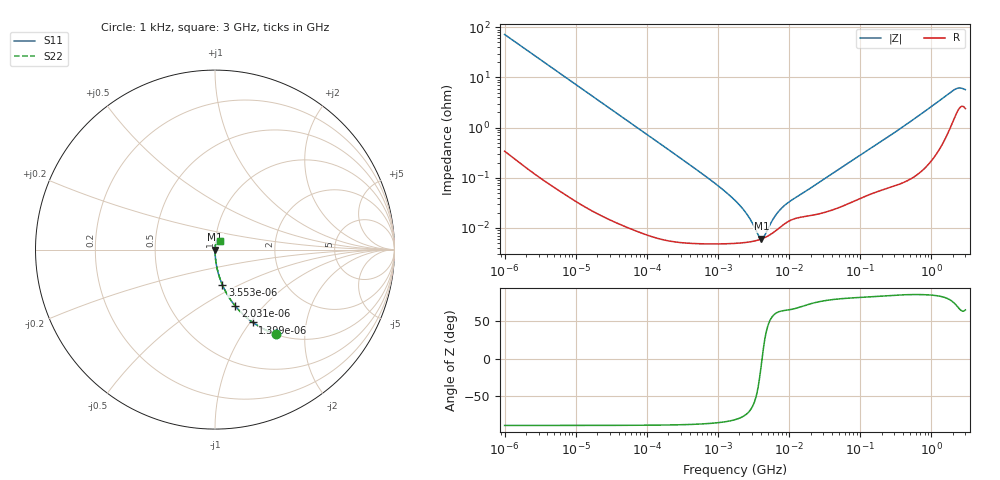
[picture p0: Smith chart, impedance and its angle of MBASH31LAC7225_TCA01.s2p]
! MBASH31LAC7225_TCA01  S-PARAMETER MODEL  ( Standard Model )
! Model Generated by TAIYO YUDEN Corporation (http://www.ty-top.com)
! Version 1.0
! TAIYO YUDEN Control No. 220601
! Copyright(c) 2016 TAIYO YUDEN CO.,LTD. All Rights Reserved.
! Product Description (link to TY-COMPAS)
! https://ds.yuden.co.jp/TYCOMPAS/or/detail?pn=MBASH31LAC7225KTCA01&u=M
! Products Name : Multilayer Ceramic Capacitors
! Characteristics :
!  Capacitance : 2.2 [uF] , Rated Voltage : 100 [V] , TCC : X7S
!  Case Size : 3.2 x 1.6 / 0.126 x 0.063 [mm/inch] , Thickness : 1.6 / 0.063 [mm/inch]
!  (Conditions: Temperature = 25 [degC] , DC Bias Voltage = 0 [V])
! External Node Assignments :
!  1  o---| |---o  2
! GND o---------o GND
! Frequency Range : 1kHz  -  3GHz  [ 401 STEP ]
# MHZ S RI R 50
! Freq[MHz].  S11 Real  S11 Imag  S21 Real  S21 Imag  S12 Real  S12 Imag  S22 Real  S22 Imag
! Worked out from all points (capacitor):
!   401 points, 1 kHz to 3 GHz, reference 50 ohm
!   read as one part in series: C = 2.21 uF near 1.077 kHz
!   lowest |Z| = 6.02 mohm at 4.083 MHz (marker M1)
!   series resonance near 4.159 MHz, so ESL is about 660 pH
!   S11 on the Smith chart (normalised r, x): 1 kHz: 1.01, -1.44; 1.399 kHz: 1.00, -1.03; 2.031 kHz: 1.00, -0.71; 3.553 kHz: 1.00, -0.41; 3 GHz: 1.05, +0.10
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0.001  0.3423 -0.4721  0.6577 0.4721  0.6577 0.4721  0.3423 -0.4721
0.001399  0.211 -0.4057  0.789 0.4057  0.789 0.4057  0.211 -0.4057
0.002031  0.1132 -0.3147  0.8868 0.3147  0.8868 0.3147  0.1132 -0.3147
0.003553  0.0405 -0.195  0.9595 0.195  0.9595 0.195  0.0405 -0.195
0.006215  0.0139 -0.1148  0.9861 0.1148  0.9861 0.1148  0.0139 -0.1148
0.01216  0.00382 -0.0594  0.9962 0.0594  0.9962 0.0594  0.00382 -0.0594
0.147855  8.47e-05 -0.00493  0.9999 0.00493  0.9999 0.00493  8.47e-05 -0.00493
0.791611  4.84e-05 -0.00089  1 0.00089  1 0.00089  4.84e-05 -0.00089
1.732051  4.89e-05 -0.000349  1 0.000349  1 0.000349  4.89e-05 -0.000349
2.422679  5.09e-05 -0.0002  0.9999 0.0002  0.9999 0.0002  5.09e-05 -0.0002
3.264662  5.46e-05 -8.61e-05  0.9999 8.61e-05  0.9999 8.61e-05  5.46e-05 -8.61e-05
3.517417  5.6e-05 -5.92e-05  0.9999 5.92e-05  0.9999 5.92e-05  5.6e-05 -5.92e-05
4.083148  5.99e-05 -6.44e-06  0.9999 6.44e-06  0.9999 6.44e-06  5.99e-05 -6.44e-06
4.739869  6.56e-05 4.6e-05  0.9999 -4.6e-05  0.9999 -4.6e-05  6.56e-05 4.6e-05
5.106836  6.94e-05 7.23e-05  0.9999 -7.23e-05  0.9999 -7.23e-05  6.94e-05 7.23e-05
6.629817  8.96e-05 0.000164  0.9999 -0.000164  0.9999 -0.000164  8.96e-05 0.000164
8.291982  0.000115 0.00024  0.9999 -0.00024  0.9999 -0.00024  0.000115 0.00024
21.06097  0.000178 0.000627  0.9998 -0.000627  0.9998 -0.000627  0.000178 0.000627
256.0921  0.000676 0.00673  0.9993 -0.00673  0.9993 -0.00673  0.000676 0.00673
1990.675  0.0154 0.0513  0.9846 -0.0513  0.9846 -0.0513  0.0154 0.0513
2398.636  0.0254 0.0544  0.9746 -0.0544  0.9746 -0.0544  0.0254 0.0544
3000  0.0258 0.0494  0.9742 -0.0494  0.9742 -0.0494  0.0258 0.0494
